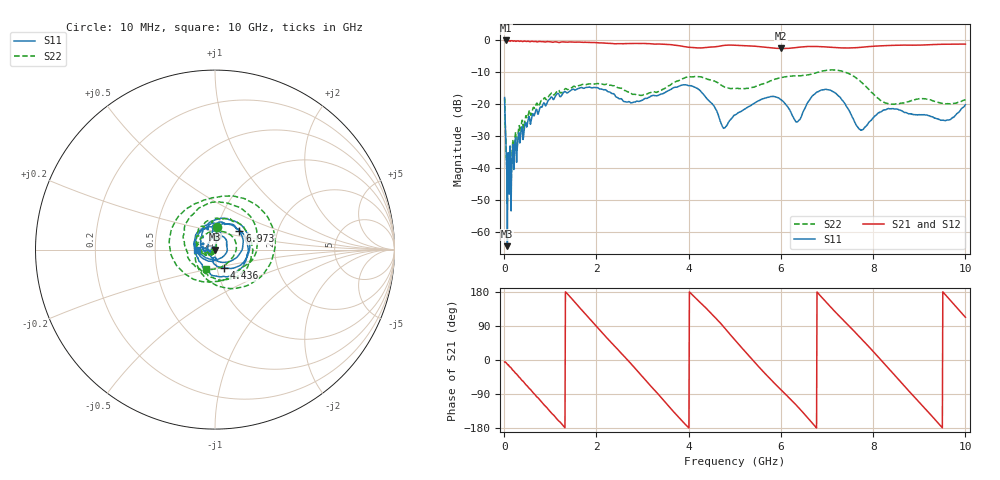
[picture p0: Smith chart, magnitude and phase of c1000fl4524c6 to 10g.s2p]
!Agilent Technologies,N5234A,MY52241123,A.10.00.00
!Agilent N5234A: A.10.00.00
!Date: Tuesday, April 16, 2019 15:12:54
!Correction: S11(Full 2 Port(1,2))
!S21(Full 2 Port(1,2))
!S12(Full 2 Port(1,2))
!S22(Full 2 Port(1,2))
!S2P File: Measurements: S11, S21, S12, S22:
# Hz S  dB  R 50
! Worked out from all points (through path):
!   1001 points, 10 MHz to 10 GHz, reference 50 ohm
!   highest |S21| = -0.05 dB at 29.98 MHz (marker M1); lowest = -2.6 dB at 6.004 GHz (marker M2)
!   group delay of S21, straight-line fit = 366 ps
!   lowest |S11| = -64.4 dB at 69.94 MHz (marker M3), VSWR 1.00, Z = 50 - j0.0592 ohm
!   |S11| at or under -10 dB: start of sweep to end of sweep
!   |S22| runs from -51.0 to -9.2 dB; largest |S21 - S12| = 0.0023
!   S11 on the Smith chart (normalised r, x): 10 MHz: 0.98, +0.25; 4.436 GHz: 1.08, -0.23; 6.973 GHz: 1.28, +0.27; 10 GHz: 0.82, -0.00
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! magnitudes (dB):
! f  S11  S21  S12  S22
! 10 MHz  -17.9  -0.1  0.0  -18.0
! 29.98 MHz  -28.5  0.0  0.0  -28.5
! 69.94 MHz  -64.4  -0.1  -0.1  -51.0
! 109.9 MHz  -48.1  -0.1  -0.1  -44.0
! 349.7 MHz  -31.3  -0.3  -0.3  -28.9
! 669.3 MHz  -22.8  -0.4  -0.3  -21.2
! 1.678 GHz  -14.8  -0.6  -0.6  -13.9
! 2.747 GHz  -19.6  -1.0  -1.0  -16.4
! 3.347 GHz  -17.2  -1.2  -1.2  -16.0
! 3.926 GHz  -13.9  -2.0  -2.0  -11.7
! 4.436 GHz  -18.8  -2.1  -2.2  -12.3
! 4.755 GHz  -27.6  -1.6  -1.6  -14.4
! 5.005 GHz  -23.3  -1.5  -1.5  -15.1
! 6.004 GHz  -18.6  -2.6  -2.6  -11.7
! 6.354 GHz  -25.5  -2.2  -2.2  -11.1
! 6.673 GHz  -17.5  -1.9  -1.9  -10.5
! 6.973 GHz  -15.3  -2.1  -2.1  -9.4
! 7.303 GHz  -18.2  -2.4  -2.4  -9.6
! 7.732 GHz  -28.1  -2.2  -2.2  -13.0
! 8.342 GHz  -21.4  -1.6  -1.6  -19.9
! 9.58 GHz  -25.0  -1.2  -1.2  -19.9
! 10 GHz  -20.2  -1.2  -1.2  -18.5
